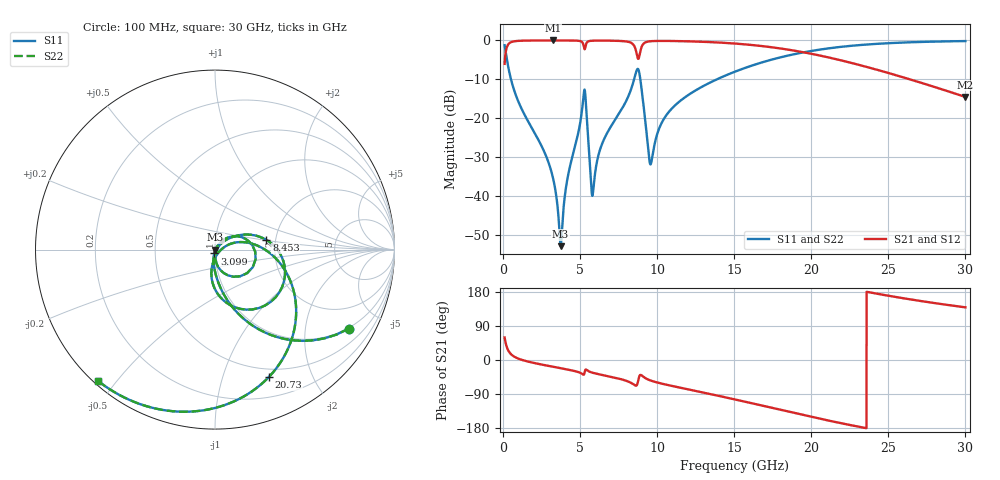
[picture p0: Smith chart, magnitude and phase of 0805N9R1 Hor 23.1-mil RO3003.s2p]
# GHz S MA R 50
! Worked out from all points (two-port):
!   3201 points, 100 MHz to 30 GHz, reference 50 ohm
!   highest |S21| = -0.02 dB at 3.249 GHz (marker M1); lowest = -14.5 dB at 30 GHz (marker M2)
!   |S21| within 3 dB of the highest: 173.1 MHz to 8.648 GHz (8.475 GHz wide, 192 % of centre); 8.893 GHz to 19.44 GHz (10.55 GHz wide, 74.5 % of centre)
!   lowest |S11| = -52.9 dB at 3.735 GHz (marker M3), VSWR 1.00, Z = 50.2 - j0.101 ohm
!   |S11| at or under -10 dB: 513.3 MHz to 8.503 GHz (7.989 GHz wide, 177 % of centre); 8.907 GHz to 13.88 GHz (4.971 GHz wide, 43.6 % of centre)
!   |S22| runs from -52.9 to -0.2 dB; largest |S21 - S12| = 0
!   S11 on the Smith chart (normalised r, x): 100 MHz: 0.97, -3.41; 3.099 GHz: 0.99, -0.04; 8.453 GHz: 1.79, +0.21; 20.73 GHz: 0.41, -1.43; 30 GHz: 0.01, -0.45
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0.1  0.8662 -30.5  0.4993 59.4  0.4993 59.4  0.8662 -30.5
0.361625  0.4301 -66.6  0.9022 23.4  0.9022 23.4  0.4301 -66.6
0.660625  0.2486 -79.3  0.9678 10.5  0.9678 10.5  0.2486 -79.3
3.099344  0.0218 -101.8  0.9978 -16.7  0.9978 -16.7  0.0218 -101.8
3.248844  0.01676 -101.2  0.9978 -17.9  0.9978 -17.9  0.01676 -101.2
3.734719  0.002268 -26.3  0.9976 -21.6  0.9976 -21.6  0.002268 -26.3
4.173875  0.01657 55.2  0.9969 -25.0  0.9969 -25.0  0.01657 55.2
5.089563  0.1128 39.4  0.9646 -35.5  0.9646 -35.5  0.1128 39.4
5.341844  0.1932 -51.7  0.8224 -25.9  0.8224 -25.9  0.1932 -51.7
5.687563  0.01729 -71.8  0.9864 -32.0  0.9864 -32.0  0.01729 -71.8
5.827719  0.01081 -0.7  0.9907 -33.7  0.9907 -33.7  0.01081 -0.7
6.435062  0.04737 44.1  0.9934 -39.5  0.9934 -39.5  0.04737 44.1
8.453312  0.2917 10.6  0.8823 -64.1  0.8823 -64.1  0.2917 10.6
8.855094  0.3688 -64.6  0.6498 -41.6  0.6498 -41.6  0.3688 -64.6
9.546531  0.02568 -45.7  0.9742 -53.7  0.9742 -53.7  0.02568 -45.7
10.06978  0.06871 18.9  0.9843 -60.1  0.9843 -60.1  0.06871 18.9
11.58347  0.1723 13.7  0.9772 -73.9  0.9772 -73.9  0.1723 13.7
15.05  0.3964 -15.2  0.9104 -104.1  0.9104 -104.1  0.3964 -15.2
20.03956  0.7336 -60.9  0.6704 -150.3  0.6704 -150.3  0.7336 -60.9
20.731  0.7706 -67.1  0.6279 -156.5  0.6279 -156.5  0.7706 -67.1
25.01978  0.9205 -101.1  0.3803 169.5  0.3803 169.5  0.9205 -101.1
30  0.9797 -131.6  0.1875 138.9  0.1875 138.9  0.9797 -131.6
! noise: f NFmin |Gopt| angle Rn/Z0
0.1  0.000714  0.9138  0.9895  0.001825
3.417  0.006326  0.7049  19.83  0.004086
6.743  0.01415  0.7407  38.3  0.009784
10.06  0.02681  0.7963  56.06  0.02128
13.39  0.02249  0.7051  71.78  0.009977
16.7  0.02757  0.7115  86.35  0.01027
20.03  0.03527  0.7382  100  0.01149
23.35  0.04634  0.7757  113.1  0.0133
26.67  0.0631  0.8199  125.9  0.01575
30  0.09023  0.866  138.7  0.01869
